| TEXAS INSTRUMENTS INCORPORATED
| Standard Linear and Logic Group
| IBIS Model of SN74ALVC162835
| 18-BIT Universal Bus Driver with 3-state outputs
| This file contains package information for the following:
|  SSOP 56-pin (DL) package as [Component] ALVC162835B_DL
|  TSSOP 56-pin (DGG) package as [Component] ALVC162835B_DGG
|  TVSOP 56-pin (DGV) package as [Component] ALVC162835B_DGV
| This device can be powered at the following Vccs:
|  3.3 volt Vcc
|  2.5 volt Vcc
|  1.8 volt Vcc
| This file provides unique models under the [Model Selector] for each Vcc.
| For operation at a specific Vcc, select the appropriate model after each
| [Model Selector] keyword.
[IBIS Ver]   3.2
[Comment char]  |_char
[File Name]   sn74alvc162835.ibs
[File Rev]   1.1 | b_die
[Date]   April 18, 2006
[Source]   Data created from TI-SPICE simulations at TI-SLL.
[Notes]   The following is an IBIS list for the SN74ALVC162835.
   Please contact sllibis@ti.com with questions and
   comments concerning SLL IBIS models.
   - FILE REV HISTORY
   - 1.1 Release IBIS file on 08/17/06
   -As there is no power clamp diode in the Input
   Models, we removed the Pwr Clamp table data from
   those Models.
   -Non-monotonic data in pullup/pulldown due to series resistor.
[Disclaimer] Property of Texas Instruments Incorporated.  Unauthorized
   reproduction and/or distribution is strictly prohibited.
   This product is protected under copyright law.
   Created  2006, (C) Copyright  2006, Texas Instruments
   Incorporated, All Rights Reserved
   UNLESS THERE IS A SIGNED, WRITTEN AGREEMENT TO THE
   CONTRARY, TEXAS INSTRUMENTS (TI) IS PROVIDING THE IBIS
   MODELS  AND WITHOUT ANY WARRANTY, EXPRESSED OR
   IMPLIED.  TI assumes no liability for:
   1) the accuracy of the IBIS models provided to your
   company;
   2) the proper functioning of these IBIS Models in your
   design or for any resulting applications; or
   3) infringement of patents, copyrights or intellectual
   property rights resulting from your use of these IBIS
   models.
   TI provides IBIS Models as a service to our customers.
   You and your company shall not distribute, sell or give
   these models to anyone else without prior written
   permission from TI.
   TI reserves the right to make changes to our products or
   to discontinue any semiconductor product or service
   without notice, and advises our customers to obtain the
   latest version of relevant information to verify, before
   placing orders, that the information being relied on is
   current.
   Please be aware that your receipt and use of the IBIS
   information provided shall serve as acceptance of these
   terms and conditions.  If you do not accept these terms,
   you should return or destroy the IBIS models and any
   other accompanying information immediately.
| Component SN74ALVC162835_DL 56-PIN SSOP
[Component]   SN74ALVC162835_DL
[Manufacturer]   Texas Instruments, Inc.
[Package]
|   typ   min   max
R_pkg   5.500e-02   4.800e-02   6.700e-02
L_pkg   6.539e-09   4.803e-09   9.746e-09
C_pkg   8.570e-13   5.000e-13   1.351e-12
[Pin]   signal_name   model_name   R_pin   L_pin   C_pin
1   NC   NC   6.400e-02   9.646e-09   1.202e-12
2   NC   NC   5.900e-02   8.723e-09   1.348e-12
3   Y1   ALVC162835_OUT   5.900e-02   8.139e-09   1.223e-12
4   GND   GND   5.600e-02   7.554e-09   1.088e-12
5   Y2   ALVC162835_OUT   5.400e-02   6.991e-09   9.660e-13
6   Y3   ALVC162835_OUT   5.300e-02   6.659e-09   9.730e-13
7   VCC   POWER   5.500e-02   6.321e-09   9.050e-13
8   Y4   ALVC162835_OUT   5.600e-02   5.942e-09   7.130e-13
9   Y5   ALVC162835_OUT   5.700e-02   5.768e-09   6.780e-13
10   Y6   ALVC162835_OUT   5.400e-02   5.459e-09   6.310e-13
11   GND   GND   5.100e-02   5.224e-09   6.380e-13
12   Y7   ALVC162835_OUT   4.800e-02   5.088e-09   6.010e-13
13   Y8   ALVC162835_OUT   5.000e-02   5.021e-09   5.180e-13
14   Y9   ALVC162835_OUT   5.100e-02   4.803e-09   5.000e-13
15   Y10   ALVC162835_OUT   5.100e-02   4.803e-09   5.000e-13
16   Y11   ALVC162835_OUT   5.000e-02   5.021e-09   5.180e-13
17   Y12   ALVC162835_OUT   4.800e-02   5.088e-09   6.010e-13
18   GND   GND   5.100e-02   5.224e-09   6.380e-13
19   Y13   ALVC162835_OUT   5.400e-02   5.459e-09   6.310e-13
20   Y14   ALVC162835_OUT   5.700e-02   5.768e-09   6.770e-13
21   Y15   ALVC162835_OUT   5.500e-02   5.942e-09   7.150e-13
22   VCC   POWER   5.500e-02   6.321e-09   9.070e-13
23   Y16   ALVC162835_OUT   5.300e-02   6.659e-09   9.720e-13
24   Y17   ALVC162835_OUT   5.400e-02   6.991e-09   9.660e-13
25   GND   GND   5.600e-02   7.554e-09   1.087e-12
26   Y18   ALVC162835_OUT   5.900e-02   8.139e-09   1.223e-12
27   NOE   ALVC162835_CTRL   5.900e-02   8.727e-09   1.351e-12
28   LE   ALVC162835_CTRL   6.700e-02   9.746e-09   1.210e-12
29   GND   GND   6.300e-02   9.630e-09   1.203e-12
30   CLK   NC   6.000e-02   8.751e-09   1.349e-12
31   A18   ALVC162835_IN   6.000e-02   8.184e-09   1.224e-12
32   GND   GND   5.600e-02   7.543e-09   1.087e-12
33   A17   ALVC162835_IN   5.400e-02   7.005e-09   9.690e-13
34   A16   ALVC162835_IN   5.600e-02   6.714e-09   9.750e-13
35   VCC   POWER   5.800e-02   6.384e-09   9.090e-13
36   A15   ALVC162835_IN   5.700e-02   5.976e-09   7.170e-13
37   A14   ALVC162835_IN   5.700e-02   5.743e-09   6.770e-13
38   A13   ALVC162835_IN   5.400e-02   5.468e-09   6.310e-13
39   GND   GND   5.500e-02   5.329e-09   6.440e-13
40   A12   ALVC162835_IN   5.200e-02   5.189e-09   6.060e-13
41   A11   ALVC162835_IN   5.200e-02   5.053e-09   5.190e-13
42   A10   ALVC162835_IN   5.200e-02   4.825e-09   5.020e-13
43   A9   ALVC162835_IN   5.400e-02   4.897e-09   5.060e-13
44   A8   ALVC162835_IN   5.200e-02   5.093e-09   5.210e-13
45   A7   ALVC162835_IN   5.100e-02   5.179e-09   6.080e-13
46   GND   GND   5.400e-02   5.314e-09   6.450e-13
47   A6   ALVC162835_IN   5.500e-02   5.511e-09   6.320e-13
48   A5   ALVC162835_IN   5.700e-02   5.770e-09   6.770e-13
49   A4   ALVC162835_IN   5.600e-02   5.956e-09   7.160e-13
50   VCC   POWER   5.500e-02   6.320e-09   9.050e-13
51   A3   ALVC162835_IN   5.200e-02   6.621e-09   9.680e-13
52   A2   ALVC162835_IN   5.300e-02   6.974e-09   9.660e-13
53   GND   GND   5.700e-02   7.571e-09   1.089e-12
54   A1   ALVC162835_IN   5.700e-02   8.097e-09   1.219e-12
55   NC   NC   5.900e-02   8.723e-09   1.349e-12
56   GND   GND   6.100e-02   9.560e-09   1.199e-12
| Component SN74ALVC162835_DGG 56-PIN TSSOP
[Component]   SN74ALVC162835_DGG
[Manufacturer]   Texas Instruments, Inc.
[Package]
|   typ   min   max
R_pkg   5.400e-02   4.000e-02   8.300e-02
L_pkg   3.546e-09   2.838e-09   5.045e-09
C_pkg   5.580e-13   4.120e-13   7.380e-13
[Pin]   signal_name   model_name   R_pin   L_pin   C_pin
1   NC   NC   7.600e-02   5.003e-09   7.120e-13
2   NC   NC   7.600e-02   4.539e-09   7.230e-13
3   Y1   ALVC162835_OUT   8.300e-02   4.357e-09   7.080e-13
4   GND   GND   4.200e-02   3.999e-09   6.830e-13
5   Y2   ALVC162835_OUT   4.200e-02   3.806e-09   6.700e-13
6   Y3   ALVC162835_OUT   4.300e-02   3.603e-09   6.160e-13
7   VCC   POWER   4.400e-02   3.440e-09   5.520e-13
8   Y4   ALVC162835_OUT   4.600e-02   3.306e-09   5.090e-13
9   Y5   ALVC162835_OUT   4.700e-02   3.194e-09   4.820e-13
10   Y6   ALVC162835_OUT   4.800e-02   3.088e-09   4.630e-13
11   GND   GND   5.000e-02   2.987e-09   4.350e-13
12   Y7   ALVC162835_OUT   5.100e-02   2.910e-09   4.230e-13
13   Y8   ALVC162835_OUT   5.200e-02   2.894e-09   4.220e-13
14   Y9   ALVC162835_OUT   5.300e-02   2.840e-09   4.220e-13
15   Y10   ALVC162835_OUT   5.300e-02   2.850e-09   4.230e-13
16   Y11   ALVC162835_OUT   5.200e-02   2.886e-09   4.210e-13
17   Y12   ALVC162835_OUT   5.100e-02   2.883e-09   4.190e-13
18   GND   GND   5.000e-02   2.941e-09   4.300e-13
19   Y13   ALVC162835_OUT   4.900e-02   3.031e-09   4.570e-13
20   Y14   ALVC162835_OUT   4.700e-02   3.131e-09   4.760e-13
21   Y15   ALVC162835_OUT   4.600e-02   3.244e-09   5.030e-13
22   VCC   POWER   4.400e-02   3.387e-09   5.500e-13
23   Y16   ALVC162835_OUT   4.300e-02   3.566e-09   6.320e-13
24   Y17   ALVC162835_OUT   4.200e-02   3.801e-09   6.870e-13
25   GND   GND   4.100e-02   3.961e-09   6.870e-13
26   Y18   ALVC162835_OUT   8.100e-02   4.291e-09   7.110e-13
27   NOE   ALVC162835_CTRL   7.600e-02   4.561e-09   7.380e-13
28   LE   ALVC162835_CTRL   7.500e-02   5.045e-09   7.240e-13
29   GND   GND   7.300e-02   5.020e-09   7.140e-13
30   CLK   NC   7.400e-02   4.532e-09   7.200e-13
31   A18   ALVC162835_IN   8.300e-02   4.336e-09   7.080e-13
32   GND   GND   4.000e-02   3.957e-09   6.840e-13
33   A17   ALVC162835_IN   4.200e-02   3.789e-09   6.800e-13
34   A16   ALVC162835_IN   4.300e-02   3.540e-09   6.240e-13
35   VCC   POWER   4.400e-02   3.361e-09   5.460e-13
36   A15   ALVC162835_IN   4.600e-02   3.222e-09   4.980e-13
37   A14   ALVC162835_IN   4.700e-02   3.110e-09   4.710e-13
38   A13   ALVC162835_IN   4.800e-02   3.012e-09   4.510e-13
39   GND   GND   5.000e-02   2.934e-09   4.230e-13
40   A12   ALVC162835_IN   5.100e-02   2.879e-09   4.120e-13
41   A11   ALVC162835_IN   5.200e-02   2.883e-09   4.130e-13
42   A10   ALVC162835_IN   5.300e-02   2.847e-09   4.170e-13
43   A9   ALVC162835_IN   5.300e-02   2.838e-09   4.170e-13
44   A8   ALVC162835_IN   5.200e-02   2.887e-09   4.160e-13
45   A7   ALVC162835_IN   5.100e-02   2.897e-09   4.160e-13
46   GND   GND   5.000e-02   2.965e-09   4.270e-13
47   A6   ALVC162835_IN   4.800e-02   3.047e-09   4.550e-13
48   A5   ALVC162835_IN   4.700e-02   3.138e-09   4.740e-13
49   A4   ALVC162835_IN   4.600e-02   3.250e-09   5.030e-13
50   VCC   POWER   4.400e-02   3.390e-09   5.500e-13
51   A3   ALVC162835_IN   4.300e-02   3.546e-09   6.260e-13
52   A2   ALVC162835_IN   4.200e-02   3.783e-09   6.860e-13
53   GND   GND   4.000e-02   3.955e-09   6.820e-13
54   A1   ALVC162835_IN   8.300e-02   4.330e-09   7.010e-13
55   NC   NC   7.700e-02   4.562e-09   7.240e-13
56   GND   GND   7.500e-02   5.029e-09   7.120e-13
| Component SN74ALVC162835_DGV 56-PIN TVSOP
[Component]   SN74ALVC162835_DGV
[Manufacturer]   Texas Instruments, Inc.
[Package]
|   typ   min   max
R_pkg   6.300e-02   5.000e-02   8.400e-02
L_pkg   2.945e-09   2.394e-09   3.939e-09
C_pkg   3.910e-13   2.710e-13   5.880e-13
[Pin]   signal_name   model_name   R_pin   L_pin   C_pin
1   NC   NC   6.800e-02   3.933e-09   5.880e-13
2   NC   NC   6.800e-02   3.568e-09   5.870e-13
3   Y1   ALVC162835_OUT   7.600e-02   3.464e-09   5.150e-13
4   GND   GND   8.400e-02   3.444e-09   4.590e-13
5   Y2   ALVC162835_OUT   8.100e-02   3.277e-09   4.270e-13
6   Y3   ALVC162835_OUT   7.400e-02   3.136e-09   3.870e-13
7   VCC   POWER   6.900e-02   2.970e-09   4.010e-13
8   Y4   ALVC162835_OUT   5.000e-02   2.785e-09   3.790e-13
9   Y5   ALVC162835_OUT   5.100e-02   2.685e-09   3.200e-13
10   Y6   ALVC162835_OUT   5.300e-02   2.611e-09   3.160e-13
11   GND   GND   5.300e-02   2.495e-09   2.970e-13
12   Y7   ALVC162835_OUT   5.300e-02   2.435e-09   2.920e-13
13   Y8   ALVC162835_OUT   5.500e-02   2.412e-09   2.850e-13
14   Y9   ALVC162835_OUT   5.600e-02   2.401e-09   2.730e-13
15   Y10   ALVC162835_OUT   5.500e-02   2.401e-09   2.730e-13
16   Y11   ALVC162835_OUT   5.500e-02   2.399e-09   2.840e-13
17   Y12   ALVC162835_OUT   5.400e-02   2.406e-09   2.890e-13
18   GND   GND   5.300e-02   2.450e-09   2.930e-13
19   Y13   ALVC162835_OUT   5.100e-02   2.544e-09   3.110e-13
20   Y14   ALVC162835_OUT   5.100e-02   2.626e-09   3.150e-13
21   Y15   ALVC162835_OUT   5.000e-02   2.727e-09   3.690e-13
22   VCC   POWER   6.500e-02   2.903e-09   3.930e-13
23   Y16   ALVC162835_OUT   7.500e-02   3.091e-09   3.860e-13
24   Y17   ALVC162835_OUT   8.200e-02   3.272e-09   4.280e-13
25   GND   GND   8.200e-02   3.393e-09   4.570e-13
26   Y18   ALVC162835_OUT   7.300e-02   3.380e-09   5.080e-13
27   NOE   ALVC162835_CTRL   7.100e-02   3.577e-09   5.800e-13
28   LE   ALVC162835_CTRL   6.800e-02   3.937e-09   5.740e-13
29   GND   GND   6.900e-02   3.923e-09   5.690e-13
30   CLK   NC   6.400e-02   3.536e-09   5.740e-13
31   A18   ALVC162835_IN   7.600e-02   3.428e-09   5.170e-13
32   GND   GND   8.100e-02   3.395e-09   4.680e-13
33   A17   ALVC162835_IN   8.000e-02   3.255e-09   4.310e-13
34   A16   ALVC162835_IN   7.100e-02   3.064e-09   3.860e-13
35   VCC   POWER   6.100e-02   2.878e-09   3.890e-13
36   A15   ALVC162835_IN   5.000e-02   2.710e-09   3.630e-13
37   A14   ALVC162835_IN   5.000e-02   2.606e-09   3.110e-13
38   A13   ALVC162835_IN   5.200e-02   2.534e-09   3.060e-13
39   GND   GND   5.200e-02   2.439e-09   2.890e-13
40   A12   ALVC162835_IN   5.300e-02   2.399e-09   2.860e-13
41   A11   ALVC162835_IN   5.500e-02   2.394e-09   2.820e-13
42   A10   ALVC162835_IN   5.500e-02   2.398e-09   2.710e-13
43   A9   ALVC162835_IN   5.600e-02   2.396e-09   2.710e-13
44   A8   ALVC162835_IN   5.400e-02   2.402e-09   2.830e-13
45   A7   ALVC162835_IN   5.400e-02   2.423e-09   2.880e-13
46   GND   GND   5.300e-02   2.474e-09   2.920e-13
47   A6   ALVC162835_IN   5.100e-02   2.569e-09   3.090e-13
48   A5   ALVC162835_IN   5.100e-02   2.638e-09   3.130e-13
49   A4   ALVC162835_IN   5.100e-02   2.742e-09   3.660e-13
50   VCC   POWER   6.400e-02   2.917e-09   3.900e-13
51   A3   ALVC162835_IN   7.400e-02   3.083e-09   3.830e-13
52   A2   ALVC162835_IN   8.100e-02   3.249e-09   4.300e-13
53   GND   GND   8.300e-02   3.400e-09   4.550e-13
54   A1   ALVC162835_IN   7.500e-02   3.427e-09   5.050e-13
55   NC   NC   7.100e-02   3.585e-09   5.780e-13
56   GND   GND   6.900e-02   3.939e-09   5.810e-13
| Model ALVC162835_IN
[Model Selector]   ALVC162835_IN
ALVC162835_IN_33   3.3 volt Vcc
ALVC162835_IN_25   2.5 volt Vcc
ALVC162835_IN_18   1.8 volt Vcc
| Model ALVC162835_CTRL
[Model Selector]   ALVC162835_CTRL
ALVC162835_CTRL_33   3.3 volt Vcc
ALVC162835_CTRL_25   2.5 volt Vcc
ALVC162835_CTRL_18   1.8 volt Vcc
| Model ALVC162835_OUT
[Model Selector]   ALVC162835_OUT
ALVC162835_OUT_33   3.3 volt Vcc
ALVC162835_OUT_25   2.5 volt Vcc
ALVC162835_OUT_18   1.8 volt Vcc
| Models and submodels in the file (9): ALVC162835_IN_33 (Input), ALVC162835_IN_25 (Input), ALVC162835_IN_18 (Input), ALVC162835_CTRL_33 (Input), ALVC162835_CTRL_25 (Input), ALVC162835_CTRL_18 (Input), ALVC162835_OUT_33 (3-state), ALVC162835_OUT_25 (3-state), ALVC162835_OUT_18 (3-state)
